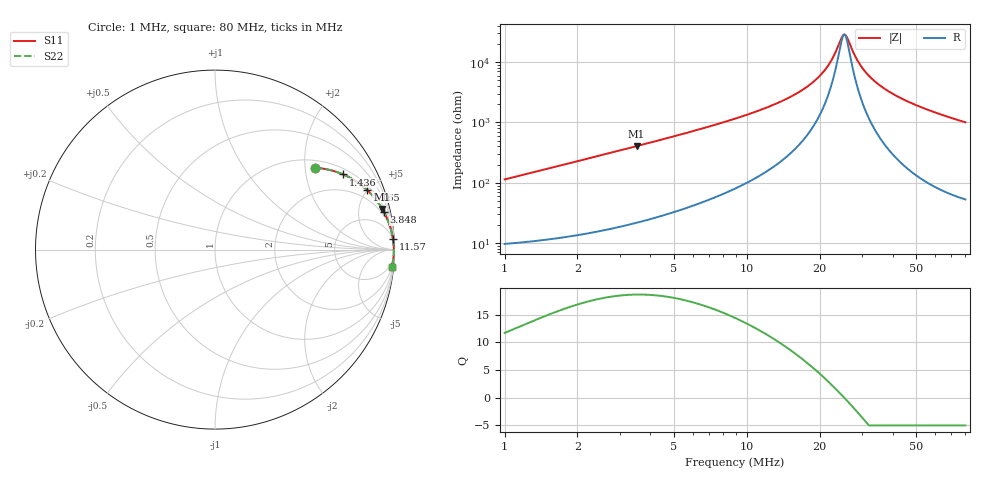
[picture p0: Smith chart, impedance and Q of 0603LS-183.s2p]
# MHz S MA R 50
!Freq  MagS11  AngS11  MagS21  AngS21  MagS12  AngS12  MagS22  AngS22
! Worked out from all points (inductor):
!   801 points, 1 MHz to 80 MHz, reference 50 ohm
!   read as one part in series: L = 18 uH near 1.022 MHz
!   highest Q = 18.6 at 3.506 MHz (marker M1), where L = 18.3 uH
!   self-resonance near 25.19 MHz
!   S11 on the Smith chart (normalised r, x): 1 MHz: 1.19, +2.26; 1.436 MHz: 1.22, +3.26; 2.165 MHz: 1.29, +4.93; 3.848 MHz: 1.48, +8.90; 11.57 MHz: 4, +33; 80 MHz: 2, -20
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1  0.7209 39.2  0.6344 -45.9  0.6344 -45.9  0.7209 39.2
1.435506  0.8278 30.4  0.5073 -55.7  0.5073 -55.7  0.8278 30.4
2.164809  0.9088 21.6  0.3681 -65.1  0.3681 -65.1  0.9088 21.6
3.505577  0.9588 13.7  0.2371 -73.2  0.2371 -73.2  0.9588 13.7
3.847691  0.9647 12.5  0.2165 -74.4  0.2165 -74.4  0.9647 12.5
6.838813  0.9858 6.8  0.1182 -79.7  0.1182 -79.7  0.9858 6.8
11.57048  0.9932 3.4  0.06018 -81.8  0.06018 -81.8  0.9932 3.4
14.16999  0.9946 2.4  0.04279 -81.5  0.04279 -81.5  0.9946 2.4
17.93331  0.9957 1.4  0.02472 -79.4  0.02472 -79.4  0.9957 1.4
20.56516  0.9962 0.8  0.01498 -74.7  0.01498 -74.7  0.9962 0.8
22.32621  0.9963 0.5  0.009427 -67.0  0.009427 -67.0  0.9963 0.5
24.50506  0.9965 0.1  0.004133 -32.1  0.004133 -32.1  0.9965 0.1
25.04789  0.9965 0.0  0.003539 -11.0  0.003539 -11.0  0.9965 0.0
25.88477  0.9966 -0.1  0.003799 25.0  0.003799 25.0  0.9966 -0.1
27.34217  0.9966 -0.3  0.006403 57.7  0.006403 57.7  0.9966 -0.3
29.5214  0.9966 -0.6  0.01131 72.3  0.01131 72.3  0.9966 -0.6
32.22544  0.9966 -1.0  0.01735 78.1  0.01735 78.1  0.9966 -1.0
35.75997  0.9964 -1.4  0.02482 81.0  0.02482 81.0  0.9964 -1.4
40.56122  0.9961 -2.0  0.03427 82.5  0.03427 82.5  0.9961 -2.0
53.9277  0.9947 -3.3  0.0579 83.1  0.0579 83.1  0.9947 -3.3
67.13769  0.9926 -4.5  0.07907 82.3  0.07907 82.3  0.9926 -4.5
80  0.99 -5.6  0.09853 81.3  0.09853 81.3  0.99 -5.6
